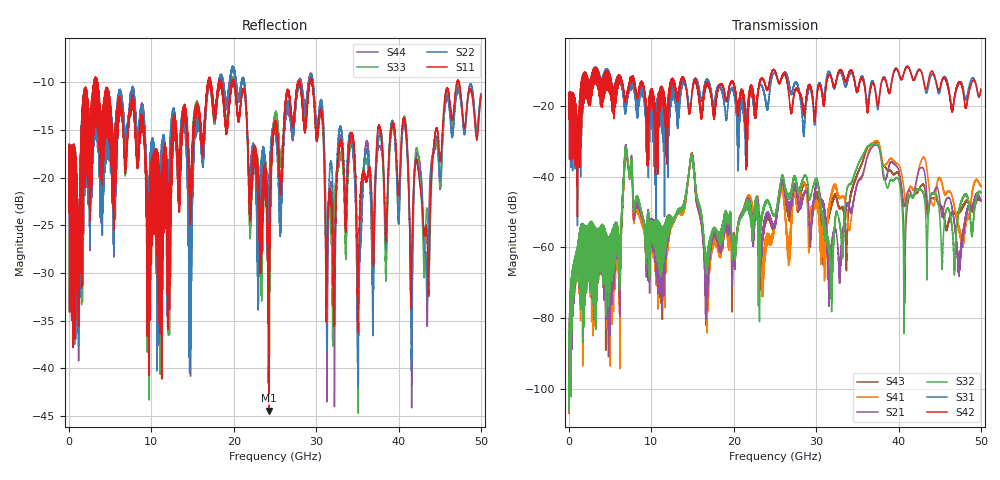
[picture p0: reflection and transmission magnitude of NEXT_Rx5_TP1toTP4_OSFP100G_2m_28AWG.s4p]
! Touchstone data
! Created: 27-Feb-2019 by IdEM 12 (12.1.0)
! COMMENTS
!  Created Wed Feb 27 12:03:36 2019
!  64 Port Network Data from SP1.SP block
!  freq  magS1_1  angS1_1  magS1_2  angS1_2  magS1_3  angS1_3  magS1_4  angS1_4
!  magS1_5  angS1_5  magS1_6  angS1_6  magS1_7  angS1_7  magS1_8  angS1_8
!  magS1_9  angS1_9  magS1_10  angS1_10  magS1_11  angS1_11  magS1_12  angS1_12
!  magS1_13  angS1_13  magS1_14  angS1_14  magS1_15  angS1_15  magS1_16  angS1_16
!  magS1_17  angS1_17  magS1_18  angS1_18  magS1_19  angS1_19  magS1_20  angS1_20
!  magS1_21  angS1_21  magS1_22  angS1_22  magS1_23  angS1_23  magS1_24  angS1_24
!  magS1_25  angS1_25  magS1_26  angS1_26  magS1_27  angS1_27  magS1_28  angS1_28
!  magS1_29  angS1_29  magS1_30  angS1_30  magS1_31  angS1_31  magS1_32  angS1_32
!  magS1_33  angS1_33  magS1_34  angS1_34  magS1_35  angS1_35  magS1_36  angS1_36
!  magS1_37  angS1_37  magS1_38  angS1_38  magS1_39  angS1_39  magS1_40  angS1_40
!  magS1_41  angS1_41  magS1_42  angS1_42  magS1_43  angS1_43  magS1_44  angS1_44
!  magS1_45  angS1_45  magS1_46  angS1_46  magS1_47  angS1_47  magS1_48  angS1_48
!  magS1_49  angS1_49  magS1_50  angS1_50  magS1_51  angS1_51  magS1_52  angS1_52
!  magS1_53  angS1_53  magS1_54  angS1_54  magS1_55  angS1_55  magS1_56  angS1_56
!  magS1_57  angS1_57  magS1_58  angS1_58  magS1_59  angS1_59  magS1_60  angS1_60
!  magS1_61  angS1_61  magS1_62  angS1_62  magS1_63  angS1_63  magS1_64  angS1_64
!  magS2_1  angS2_1  magS2_2  angS2_2  magS2_3  angS2_3  magS2_4  angS2_4
!  magS2_5  angS2_5  magS2_6  angS2_6  magS2_7  angS2_7  magS2_8  angS2_8
!  magS2_9  angS2_9  magS2_10  angS2_10  magS2_11  angS2_11  magS2_12  angS2_12
!  magS2_13  angS2_13  magS2_14  angS2_14  magS2_15  angS2_15  magS2_16  angS2_16
!  magS2_17  angS2_17  magS2_18  angS2_18  magS2_19  angS2_19  magS2_20  angS2_20
!  magS2_21  angS2_21  magS2_22  angS2_22  magS2_23  angS2_23  magS2_24  angS2_24
!  magS2_25  angS2_25  magS2_26  angS2_26  magS2_27  angS2_27  magS2_28  angS2_28
!  magS2_29  angS2_29  magS2_30  angS2_30  magS2_31  angS2_31  magS2_32  angS2_32
!  magS2_33  angS2_33  magS2_34  angS2_34  magS2_35  angS2_35  magS2_36  angS2_36
!  magS2_37  angS2_37  magS2_38  angS2_38  magS2_39  angS2_39  magS2_40  angS2_40
!  magS2_41  angS2_41  magS2_42  angS2_42  magS2_43  angS2_43  magS2_44  angS2_44
!  magS2_45  angS2_45  magS2_46  angS2_46  magS2_47  angS2_47  magS2_48  angS2_48
!  magS2_49  angS2_49  magS2_50  angS2_50  magS2_51  angS2_51  magS2_52  angS2_52
!  magS2_53  angS2_53  magS2_54  angS2_54  magS2_55  angS2_55  magS2_56  angS2_56
!  magS2_57  angS2_57  magS2_58  angS2_58  magS2_59  angS2_59  magS2_60  angS2_60
!  magS2_61  angS2_61  magS2_62  angS2_62  magS2_63  angS2_63  magS2_64  angS2_64
!  magS3_1  angS3_1  magS3_2  angS3_2  magS3_3  angS3_3  magS3_4  angS3_4
!  magS3_5  angS3_5  magS3_6  angS3_6  magS3_7  angS3_7  magS3_8  angS3_8
!  magS3_9  angS3_9  magS3_10  angS3_10  magS3_11  angS3_11  magS3_12  angS3_12
!  magS3_13  angS3_13  magS3_14  angS3_14  magS3_15  angS3_15  magS3_16  angS3_16
!  magS3_17  angS3_17  magS3_18  angS3_18  magS3_19  angS3_19  magS3_20  angS3_20
!  magS3_21  angS3_21  magS3_22  angS3_22  magS3_23  angS3_23  magS3_24  angS3_24
!  magS3_25  angS3_25  magS3_26  angS3_26  magS3_27  angS3_27  magS3_28  angS3_28
!  magS3_29  angS3_29  magS3_30  angS3_30  magS3_31  angS3_31  magS3_32  angS3_32
!  magS3_33  angS3_33  magS3_34  angS3_34  magS3_35  angS3_35  magS3_36  angS3_36
!  magS3_37  angS3_37  magS3_38  angS3_38  magS3_39  angS3_39  magS3_40  angS3_40
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# Hz S MA R 50
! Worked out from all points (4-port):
!   5000 points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, 10 MHz to 50 GHz, reference 50 ohm
!   strongest paths, dB at 10 MHz, 12.51 GHz, 25.01 GHz, 37.51 GHz, 50 GHz:
!     S42: -18.1, -13.1, -10.0, -19.7, -15.2
!     S31: -18.0, -15.9, -10.7, -20.7, -15.4
!     S32: -96.6, -51.6, -50.8, -31.0, -44.4
!     S21: -98.6, -51.5, -53.1, -31.2, -46.8
!     S41: -99.1, -52.1, -53.0, -29.9, -42.7
!     S43: -98.7, -52.1, -53.4, -30.4, -46.7
!   lowest |S11| = -44.4 dB at 24.26 GHz (marker M1), VSWR 1.01, Z = 49.6 - j0.401 ohm
!   |S11| at or under -10 dB: 3.451 GHz to 16.86 GHz (13.4 GHz wide, 132 % of centre); 20.09 GHz to 27.79 GHz (7.695 GHz wide, 32.1 % of centre); 29.5 GHz to 47.1 GHz (17.61 GHz wide, 46 % of centre)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
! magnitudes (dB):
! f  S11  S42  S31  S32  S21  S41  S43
! 10 MHz  -17.7  -18.1  -18.0  -96.6  -98.6  -99.1  -98.7
! 6.95 GHz  -17.8  -17.4  -18.5  -32.7  -32.3  -33.1  -33.4
! 11.27 GHz  -19.1  -14.6  -17.1  -54.3  -55.2  -55.9  -55.6
! 14.92 GHz  -18.6  -16.4  -16.2  -34.7  -34.8  -34.5  -34.2
! 16.72 GHz  -11.4  -13.5  -12.3  -64.9  -66.7  -69.8  -70.9
! 24.26 GHz  -44.4  -13.8  -18.3  -47.4  -50.4  -57.3  -51.7
! 50 GHz  -11.4  -15.2  -15.4  -44.4  -46.8  -42.7  -46.7
